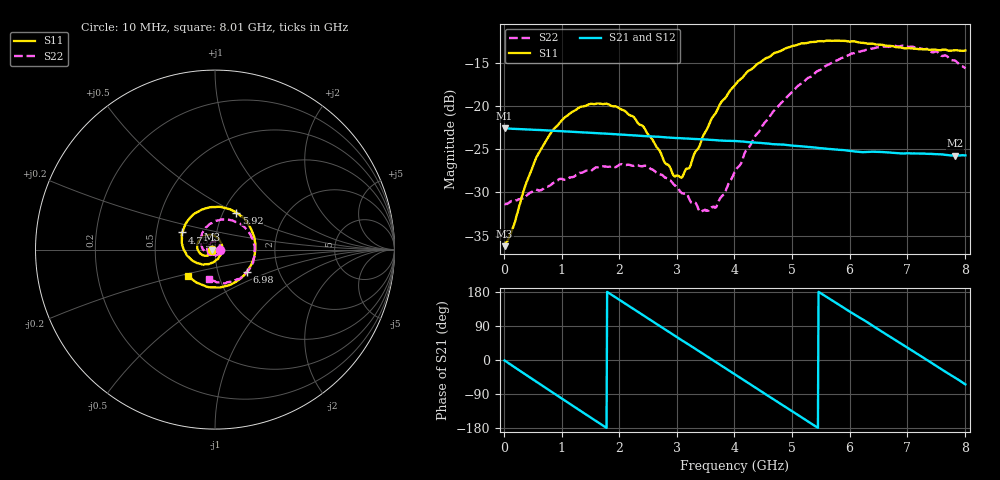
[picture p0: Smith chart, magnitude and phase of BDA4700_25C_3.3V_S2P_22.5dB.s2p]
!Agilent Technologies,E5071B,MY42404982,A.09.10
!Date: Mon Oct 20 18:12:30 2025
!Data & Calibration Information:
!Freq	S11:SOLT2(ON)	S21:SOLT2(ON)	S12:SOLT2(ON)	S22:SOLT2(ON)
# Hz S RI R 50
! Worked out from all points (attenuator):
!   801 points, 10 MHz to 8.01 GHz, reference 50 ohm
!   highest |S21| = -22.56 dB at 10 MHz (marker M1); lowest = -25.7 dB at 7.83 GHz (marker M2)
!   lowest |S11| = -36.2 dB at 10 MHz (marker M3), VSWR 1.03, Z = 48.5 - j0.115 ohm
!   |S11| at or under -10 dB: start of sweep to end of sweep
!   |S22| runs from -32.3 to -13.0 dB; largest |S21 - S12| = 0.00087
!   S11 on the Smith chart (normalised r, x): 10 MHz: 0.97, -0.00; 4.75 GHz: 0.68, +0.14; 5.92 GHz: 1.15, +0.50; 6.98 GHz: 1.38, -0.36; 8.01 GHz: 0.71, -0.22
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1e7  -0.0154 -0.00119  0.0744 -0.0016  0.0744 -0.00167  0.0271 -0.000837
6e8  -0.041 -0.034  0.0351 -0.0636  0.035 -0.0636  0.0131 -0.0297
1.01e9  -0.0797 -0.0243  -0.0153 -0.0698  -0.0153 -0.0698  -0.0155 -0.0345
1.35e9  -0.099 0.00831  -0.051 -0.0486  -0.0511 -0.0486  -0.0369 -0.018
2.08e9  -0.0483 0.0811  -0.0597 0.033  -0.0597 0.033  -0.0298 0.0345
2.42e9  -0.000285 0.076  -0.031 0.0595  -0.031 0.0595  -0.00427 0.0447
2.68e9  0.0285 0.0486  -0.00234 0.0663  -0.0024 0.0662  0.0139 0.038
2.95e9  0.0387 0.00732  0.027 0.0596  0.0269 0.0594  0.0264 0.0231
3.09e9  0.0354 -0.0154  0.0403 0.051  0.0399 0.0513  0.0289 0.0118
3.41e9  0.0036 -0.0604  0.0601 0.0227  0.0601 0.0227  0.0212 -0.0121
3.54e9  -0.0169 -0.0735  0.0632 0.00891  0.0633 0.00871  0.0137 -0.0206
3.7e9  -0.0487 -0.0809  0.0628 -0.00838  0.0628 -0.00852  -0.000386 -0.0269
4.01e9  -0.1135 -0.0682  0.0494 -0.0386  0.0494 -0.0385  -0.0322 -0.0265
4.75e9  -0.182 0.0954  -0.0212 -0.0561  -0.0209 -0.0562  -0.0794 0.0583
5.35e9  -0.0638 0.226  -0.0568 -0.0107  -0.0567 -0.011  -0.0157 0.1483
5.92e9  0.1194 0.2065  -0.0396 0.0388  -0.0397 0.0386  0.1136 0.1553
6.37e9  0.2134 0.0854  -0.0032 0.0543  -0.00346 0.054  0.1991 0.0795
6.68e9  0.2214 -0.0252  0.0241 0.0481  0.0243 0.048  0.2201 -0.00154
6.98e9  0.1775 -0.1231  0.0435 0.0306  0.0436 0.0302  0.2059 -0.0821
7.44e9  0.0374 -0.2088  0.052 -0.00869  0.052 -0.00867  0.1136 -0.1699
7.83e9  -0.0991 -0.1858  0.0355 -0.0375  0.0354 -0.0376  0.011 -0.183
8.01e9  -0.1498 -0.1469  0.0224 -0.0467  0.0227 -0.0466  -0.0326 -0.1618
